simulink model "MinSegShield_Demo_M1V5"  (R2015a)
settings: Solver=ode45  StartTime=0.0  StopTime=10.0  RelTol=1e-3
libraries: arduinolib x3, MinSegLibrary_M1V4 x2, RASPlib x2

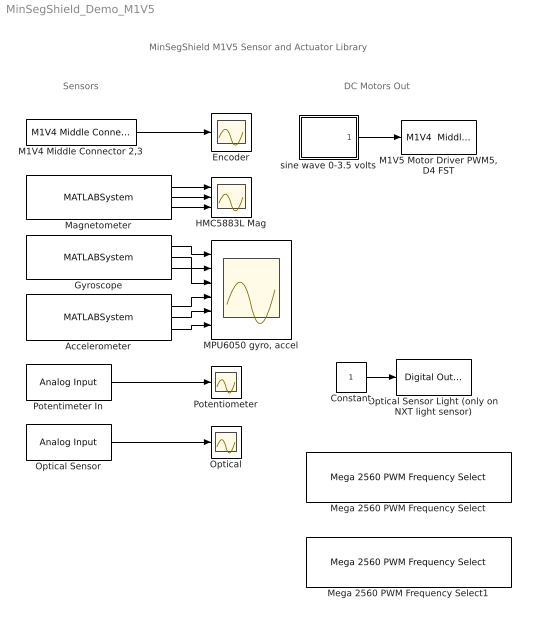
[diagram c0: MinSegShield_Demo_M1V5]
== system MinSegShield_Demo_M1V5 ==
  note: DC Motors Out
  note: Sensors
  note: MinSegShield M1V5 Sensor and Actuator Library
  Accelerometer : MATLABSystem  System=soMPU6050Accel  SimulateUsing=Code generation
  Constant : Constant
  Encoder : Scope
  Gyroscope : MATLABSystem  System=soMPU6050Gyro  DLPFmode=0
  HMC5883L Mag : Scope  NumInputPorts=3
  M1V4 Middle Connector 2,3 : MinSegLibrary_M1V4/M1V4 Middle Connector 2,3  Encoder=0  PinA=2  PinB=3  PWMFSelect=1  PWMTimer=3
  "M1V5 Motor Driver PWM5, D4 FST" : MinSegLibrary_M1V4/M1V4  Middle Motor Driver PWM5, D4 FST  Vsupply=3.5
  "MPU6050 gyro, accel" : Scope  NumInputPorts=6
  Magnetometer : MATLABSystem  System=soHMC5883L  SimulateUsing=Code generation
  Mega 2560 PWM Frequency Select : RASPlib/Mega 2560 PWM Frequency Select  Frequency=490Hz  Timer=3 - pins 2, 3, 5
  Mega 2560 PWM Frequency Select1 : RASPlib/Mega 2560 PWM Frequency Select  Frequency=32KHz  Timer=4 - pins 6, 7, 8
  Optical : Scope
  Optical Sensor : arduinolib/Analog Input  pinNumber=1  sampleTime=-1  blockPlatform=arduino
  Optical Sensor Light (only on NXT light sensor) : arduinolib/Digital Output  pinNumber=12  blockPlatform=arduino
  Potentimeter In : arduinolib/Analog Input  pinNumber=0  sampleTime=-1  blockPlatform=arduino
  Potentiometer : Scope
  sine wave 0-3.5 volts : Subsystem
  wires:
  sine wave 0-3.5 volts/1(sine) -> "M1V5 Motor Driver PWM5, D4 FST"/1
  Potentimeter In/1 -> Potentiometer/1
  Optical Sensor/1 -> Optical/1
  Constant/1 -> Optical Sensor Light (only on NXT light sensor)/1
  M1V4 Middle Connector 2,3/1 -> Encoder/1
  Gyroscope/1 -> "MPU6050 gyro, accel"/1
  Gyroscope/2 -> "MPU6050 gyro, accel"/2
  Gyroscope/3 -> "MPU6050 gyro, accel"/3
  Accelerometer/1 -> "MPU6050 gyro, accel"/4
  Accelerometer/2 -> "MPU6050 gyro, accel"/5
  Accelerometer/3 -> "MPU6050 gyro, accel"/6
  Magnetometer/1 -> HMC5883L Mag/1
  Magnetometer/2 -> HMC5883L Mag/2
  Magnetometer/3 -> HMC5883L Mag/3

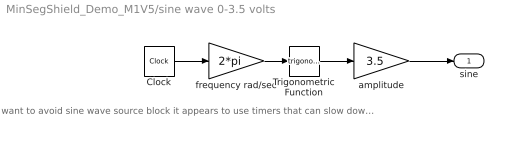
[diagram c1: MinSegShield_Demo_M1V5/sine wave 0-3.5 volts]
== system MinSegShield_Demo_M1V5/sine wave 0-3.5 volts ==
  note: want to avoid sine wave source block it appears to use timers that can slow down the serial port data transimission, and maybe other timers use a clock instead like this
  Clock : Clock
  Trigonometric Function : Trigonometry
  amplitude : Gain  Gain=3.5
  frequency rad/sec : Gain  Gain=2*pi
  sine : Outport
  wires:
  Clock/1 -> frequency rad/sec/1
  Trigonometric Function/1 -> amplitude/1
  frequency rad/sec/1 -> Trigonometric Function/1
  amplitude/1 -> sine/1
